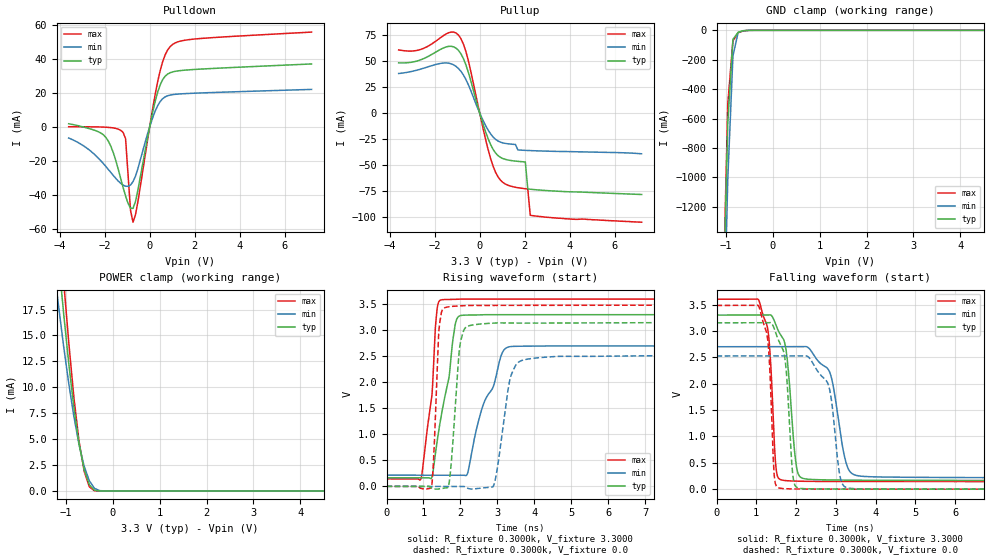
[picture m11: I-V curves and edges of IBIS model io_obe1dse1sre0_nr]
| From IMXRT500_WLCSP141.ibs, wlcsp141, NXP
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[Model] io_obe1dse1sre0_nr
|   Model io_obe1dse1sre0_nr
| Library cells for typ/min/max conditions are connected as defined below:
|  pad - External Pad
|  ipp_do - Core Input
|  ipp_obe - Output Buffer Enable
|  REFH3V3 - vdd1v8
|  REFL3V3 - REFL3V3
|  gnde - gnde
|  ipp_dse - vdd
|  ipp_ina235_3v - NC
|  ipp_ina40_3v - NC
|  ipp_ina_mux - NC
|  ipp_ind - NC
|  ipp_ind_1p8v - NC
|  ipp_ind_3v - NC
|  vdd - vdd
|  vdd1v8 - vdd1v8
|  vdda - vdde3v3
|  vdde3v3 - vdde3v3
| All other pins connected to ground
Model_type I/O
Polarity   Non-Inverting
Enable   Active-High
Vinl =   0.9900V
Vinh =   2.3100V
Vmeas =  1.6500V
Cref =   25.0000pF
Rref =   0.5000k
Vref =   0.0V
C_comp   1.8909pF   1.8218pF   2.0891pF
[Temperature Range]   25.0000   0.1250k   -40.0000
[Voltage Range]   3.3000V   2.7000V   3.6000V
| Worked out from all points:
|   slope of the pulldown table from 0 to 0.495 V, typ, clamps not added: 19.4 ohm
|   slope of the pullup table from 0 to 0.495 V, typ, clamps not added: 16 ohm
|   GND clamp passes 1 mA (typ) near -0.55 V on its own axis
|   POWER clamp passes 1 mA (typ) near -0.53 V on its own axis
|   rising waveform, R_fixture 0.3000k, V_fixture 3.3000: 20-80 % time 417ps typ, 673ps min, 255ps max; typ from 0.165 V to 3.3 V
|   rising waveform, R_fixture 0.3000k, V_fixture 0.0: 20-80 % time 186ps typ, 298ps min, 115ps max; typ from 0 V to 3.15 V
|   falling waveform, R_fixture 0.3000k, V_fixture 3.3000: 20-80 % time 212ps typ, 339ps min, 147ps max; typ from 3.3 V to 0.165 V
|   falling waveform, R_fixture 0.3000k, V_fixture 0.0: 20-80 % time 169ps typ, 264ps min, 125ps max; typ from 3.15 V to 0 V
[Pulldown]
|Voltage   I(typ)   I(min)   I(max)
-3.6V     1.86mA     -6.52mA    100uA
-1.95V    -6.13mA    -23.21mA   -180uA
-1.62V    -14.97mA   -28.49mA   -590uA
-1.18V    -35.64mA   -34.24mA   -3.216mA
-1.07V    -40.67mA   -34.88mA   -6.929mA
-850mV    -47.74mA   -34.14mA   -49.09mA
-740mV    -47.9mA    -32.2mA    -56.02mA
-520mV    -36.89mA   -24.41mA   -43.8mA
360mV     20.57mA    12.57mA    26.82mA
580mV     27.83mA    16.63mA    38.42mA
910mV     31.85mA    18.72mA    47.2mA
7.2V      37.02mA    22.05mA    55.76mA
[Pullup]
|Voltage   I(typ)   I(min)   I(max)
-3.6V     48.16mA    37.9mA     60.62mA
-2.59V    51.35mA    42.34mA    61.31mA
-1.6V     62.63mA    48.02mA    74.55mA
-940mV    60.15mA    42.71mA    74.92mA
-500mV    38.89mA    26.95mA    50.05mA
160mV     -11.43mA   -7.699mA   -15.76mA
600mV     -35.24mA   -23.3mA    -51.47mA
1.04V     -44.06mA   -28.96mA   -67.12mA
2.03V     -47.27mA   -36.13mA   -73.08mA
2.14V     -73.27mA   -36.24mA   -73.35mA
2.25V     -73.54mA   -36.34mA   -98.66mA
7.2V      -78.63mA   -39.43mA   -105.3mA
[GND_clamp]
|Voltage   I(typ)   I(min)   I(max)
-3.6V     -46.64A    -46.27A    -48.09A
-1.07V    -2.038A    -2.424A    -1.965A
-960mV    -629.9mA   -1.012A    -499.2mA
-850mV    -61.62mA   -174.1mA   -72.03mA
-740mV    -13.6mA    -15.68mA   -16.3mA
-630mV    -2.659mA   -3.244mA   -3.911mA
-410mV    -9.214uA   -49.17uA   -3.123uA
7.2V      0A         0A         0A
[POWER_clamp]
|Voltage   I(typ)   I(min)   I(max)
-3.6V     124.7mA    103.4mA    137.3mA
-1.27V    28.14mA    22.17mA    33.67mA
-1.16V    22.5mA     17.97mA    26.85mA
-1.05V    17.19mA    14.01mA    20.36mA
-940mV    12.34mA    10.39mA    14.37mA
-830mV    8.067mA    7.189mA    9.044mA
-720mV    4.554mA    4.475mA    4.783mA
-610mV    2.051mA    2.374mA    1.895mA
-500mV    596.8uA    974uA      390.7uA
-390mV    63.25uA    246uA      14.24uA
-170mV    55.4nA     1.772uA    16.57nA
7.2V      0A         0A         0A
[Ramp]
| variable   typ   min   max
dV/dt_r  1.3314/0.5971n   0.8903/1.0700n   1.7299/0.2787n
dV/dt_f  1.0033/0.3501n   0.5900/0.5957n   1.4811/0.2372n
R_load = 50.0000
[Rising Waveform]
R_fixture= 0.3000k
V_fixture= 3.3000
V_fixture_min= 2.7000
V_fixture_max= 3.6000
|time   V(typ)   V(min)   V(max)
0s        164.8mV    215.1mV    143.9mV
923.2ps   164.8mV    215.1mV    133.3mV
1.224ns   167.8mV    215.1mV    1.699V
1.395ns   987mV      215.1mV    3.51V
1.858ns   3.099V     215.1mV    3.594V
2.012ns   3.284V     215.1mV    3.599V
2.194ns   3.293V     249.4mV    3.6V
3.151ns   3.299V     2.589V     3.599V
4.14ns    3.299V     2.699V     3.6V
500ns     3.3V       2.7V       3.6V
[Rising Waveform]
R_fixture= 0.3000k
V_fixture= 0.0
V_fixture_min= 0.0
V_fixture_max= 0.0
|time   V(typ)   V(min)   V(max)
0s        31.94nV    709.3nV    82.55nV
1.215ns   -30.52mV   679.4nV    -19.82mV
1.424ns   -49.73mV   545.6nV    3.04V
1.669ns   -13.68mV   162.4nV    3.45V
1.979ns   2.663V     -23.96uV   3.47V
2.178ns   3.071V     -29.87mV   3.478V
2.902ns   3.139V     17.92mV    3.477V
3.507ns   3.138V     2.336V     3.478V
4.688ns   3.141V     2.499V     3.48V
500ns     3.153V     2.524V     3.483V
[Falling Waveform]
R_fixture= 0.3000k
V_fixture= 3.3000
V_fixture_min= 2.7000
V_fixture_max= 3.6000
|time   V(typ)   V(min)   V(max)
0s        3.3V       2.7V       3.6V
1.062ns   3.3V       2.7V       3.581V
1.411ns   3.26V      2.7V       1.613V
1.548ns   3.011V     2.7V       220.8mV
1.756ns   2.605V     2.7V       161mV
2.028ns   358.2mV    2.7V       151.6mV
2.412ns   183mV      2.583V     147.4mV
3.361ns   170.7mV    329.1mV    144.6mV
5.028ns   166.2mV    224.2mV    143.9mV
500ns     164.8mV    215.1mV    143.9mV
[Falling Waveform]
R_fixture= 0.3000k
V_fixture= 0.0
V_fixture_min= 0.0
V_fixture_max= 0.0
|time   V(typ)   V(min)   V(max)
0s        3.153V     2.524V     3.483V
1.076ns   3.153V     2.524V     3.44V
1.297ns   3.154V     2.524V     2.77V
1.419ns   3.103V     2.524V     710.7mV
1.711ns   2.522V     2.524V     9.521mV
2.079ns   18.43mV    2.524V     2.934mV
2.811ns   2.523mV    1.983V     676.8uV
3.167ns   1.632mV    98.69mV    362.9uV
3.847ns   822.1uV    4.261mV    116.2uV
500ns     406.7nV    1.167uV    330.9nV
